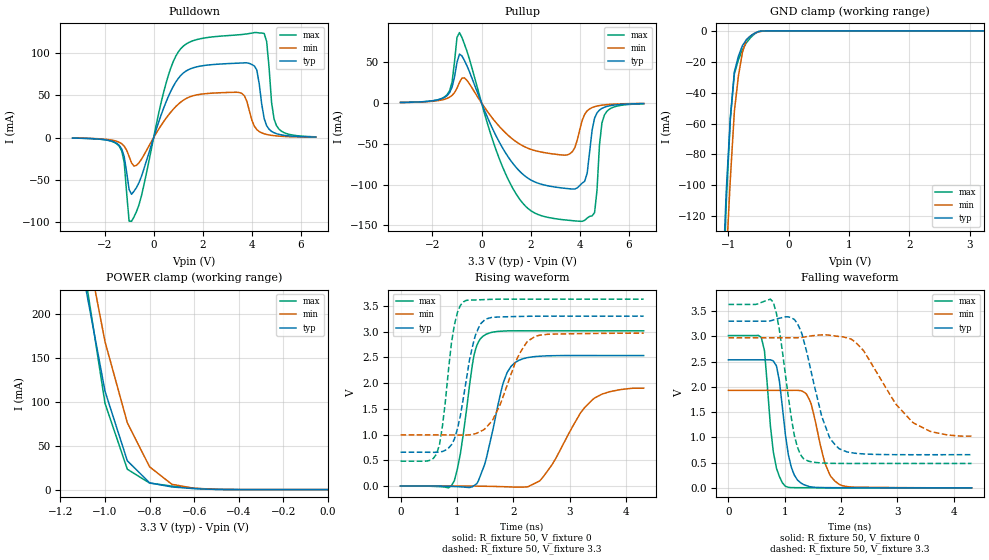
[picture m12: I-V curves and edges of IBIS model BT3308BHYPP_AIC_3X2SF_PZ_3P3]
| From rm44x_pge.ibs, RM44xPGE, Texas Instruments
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|   Model Cell BT3308BHYPP_AIC_3X2SF_PZ_3P3
|BT3308BHYPP_AIC_3X2SF_PZ_3P3
[Model]   BT3308BHYPP_AIC_3X2SF_PZ_3P3
Model_type   I/O
Polarity   Non-Inverting
Enable   Active-Low
Vinl =  1.15
Vinh =  1.55
Cref =  15.0001pF
Rref =  101.0000M
Vref =  0V
Vmeas =  1.65
C_comp   1.2p   1.2p   1.2p
[Model Spec]
Vinl   1.15   1.02   1.28
Vinh   1.55   1.45   1.65
[Temperature Range]   25   155   -40
[Voltage Range]   3.3   2.97   3.63
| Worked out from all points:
|   slope of the pulldown table from 0 to 0.495 V, typ, clamps not added: 11.9 ohm
|   slope of the pullup table from 0 to 0.495 V, typ, clamps not added: 14.3 ohm
|   GND clamp passes 1 mA (typ) near -0.53 V on its own axis
|   POWER clamp passes 1 mA (typ) near -0.59 V on its own axis
|   rising waveform, R_fixture 50, V_fixture 0: 20-80 % time 315ps typ, 599ps min, 226ps max; typ from 0 V to 2.53 V
|   rising waveform, R_fixture 50, V_fixture 3.3: 20-80 % time 265ps typ, 431ps min, 200ps max; typ from 0.657 V to 3.3 V
|   falling waveform, R_fixture 50, V_fixture 0: 20-80 % time 182ps typ, 257ps min, 153ps max; typ from 2.53 V to 0 V
|   falling waveform, R_fixture 50, V_fixture 3.3: 20-80 % time 362ps typ, 700ps min, 238ps max; typ from 3.3 V to 0.657 V
[POWER_clamp]
|   voltage   I(typ)   I(min)   I(max)
-3.3V     4.054A     4.63A      4.887A
-1.1V     248.3mA    301mA      262.7mA
-1.067V   202.9mA    256.9mA    207.9mA
-1.033V   157.5mA    212.7mA    153.1mA
-1V       112.1mA    168.6mA    98.29mA
-900mV    32.88mA    76.23mA    23.22mA
-800mV    7.705mA    25.95mA    7.475mA
-700mV    3.033mA    6.039mA    3.99mA
-600mV    1.087mA    1.528mA    1.425mA
-500mV    187uA      368.9uA    203.4uA
0V        443pA      6.158nA    417pA
[Pulldown]
|   voltage   I(typ)   I(min)   I(max)
-3.3V     -593uA     -522.6uA   -580.3uA
-1.4V     -9.188mA   -5.565mA   -10.35mA
-1.2V     -22.55mA   -10.08mA   -29.13mA
-1V       -61.66mA   -22.23mA   -99.07mA
-900mV    -67.21mA   -30.1mA    -99.29mA
1V        70.16mA    39.61mA    101.5mA
3.5V      88.44mA    53.41mA    122.1mA
4.2V      80.27mA    9.542mA    124.6mA
4.6V      14.18mA    3.749mA    114.2mA
4.8V      7.418mA    2.695mA    42.04mA
5V        4.687mA    2.03mA     14.29mA
6.6V      680.4uA    493.7uA    947.4uA
[Pullup]
|   voltage   I(typ)   I(min)   I(max)
-3.3V     671.9uA    618.2uA    613.1uA
-1.4V     9.171mA    5.687mA    10.35mA
-900mV    59.98mA    25.21mA    86.36mA
600mV     -40.93mA   -24.46mA   -58.45mA
1.4V      -78.76mA   -47.34mA   -111.2mA
3.5V      -105mA     -63.56mA   -143.7mA
4.1V      -98.16mA   -21.1mA    -145.1mA
4.3V      -85.91mA   -9.61mA    -141.1mA
4.6V      -18.69mA   -4.516mA   -134.6mA
4.8V      -8.691mA   -3.128mA   -51.49mA
5V        -5.242mA   -2.297mA   -14.81mA
6.6V      -711.8uA   -541.3uA   -921.2uA
[GND_clamp]
|   voltage   I(typ)   I(min)   I(max)
-3.3V     -3.25A     -2.875A    -4.945A
-1.1V     -166.9mA   -205mA     -187mA
-1.033V   -102.7mA   -146.7mA   -110.1mA
-966.7mV  -55.96mA   -95.69mA   -57.01mA
-900mV    -26.55mA   -52.03mA   -27.79mA
-833.3mV  -16.49mA   -29.28mA   -18.76mA
-766.7mV  -9.537mA   -13.91mA   -12.06mA
-700mV    -5.687mA   -5.923mA   -7.702mA
-566.7mV  -1.566mA   -1.63mA    -2.054mA
-500mV    -402.1uA   -594uA     -459.6uA
-366.7mV  -18.7uA    -59.22uA   -17.4uA
3.233V    423.5pA    4.09uA     323pA
[Ramp]
| variable   typ   min   max
dV/dt_f   1.638302/0.3729057n   1.223267/0.733161n   1.953849/0.2452135n
dV/dt_r   1.540285/0.3180453n   1.172218/0.6246788n   1.831658/0.2269715n
R_load = 50
[Rising Waveform]
R_fixture = 50
V_fixture = 0
V_fixture_min = 0
V_fixture_max = 0
|   time   V(typ)   V(min)   V(max)
0s        -4.976uV   -2.78uV    -6.755uV
956ps     -9.91mV    198.9uV    105mV
1.064ns   -15.38mV   128.6uV    636mV
1.304ns   7.149mV    -1.954mV   2.538V
1.492ns   414.2mV    -4.662mV   2.929V
1.82ns    1.995V     -12.79mV   3.009V
2.036ns   2.4V       -21.33mV   3.015V
2.472ns   2.521V     99.87mV    3.014V
3.444ns   2.534V     1.708V     3.014V
4.316ns   2.534V     1.9V       3.014V
[Rising Waveform]
R_fixture = 50
V_fixture = 3.3
V_fixture_min = 2.97
V_fixture_max = 3.63
|   time   V(typ)   V(min)   V(max)
0s        656.6mV    993.3mV    482.4mV
640ps     655.6mV    993.3mV    623.4mV
744ps     671mV      993.1mV    1.162V
956ps     911.4mV    990.3mV    3.129V
1.116ns   1.712V     987.9mV    3.576V
1.332ns   2.938V     1.017V     3.614V
1.52ns    3.244V     1.138V     3.622V
2.108ns   3.294V     2.562V     3.63V
2.4ns     3.298V     2.911V     3.63V
4.316ns   3.3V       2.969V     3.63V
[Falling Waveform]
R_fixture = 50
V_fixture = 0
V_fixture_min = 0
V_fixture_max = 0
|   time   V(typ)   V(min)   V(max)
0s        2.534V     1.93V      3.014V
584ps     2.533V     1.93V      2.975V
640ps     2.533V     1.93V      2.71V
852ps     2.415V     1.93V      389.6mV
1.012ns   1.045V     1.93V      30.07mV
1.224ns   156.7mV    1.93V      3.731mV
1.44ns    23.5mV     1.74V      1.968mV
1.712ns   5.245mV    492.9mV    537.2uV
1.964ns   2.809mV    70.58mV    297.7uV
4.316ns   94.61uV    817.4uV    5.461uV
[Falling Waveform]
R_fixture = 50
V_fixture = 3.3
V_fixture_min = 2.97
V_fixture_max = 3.63
|   time   V(typ)   V(min)   V(max)
0s        3.3V       2.97V      3.63V
796ps     3.322V     2.97V      3.674V
904ps     3.358V     2.97V      3.127V
1.168ns   3.334V     2.97V      1.044V
1.332ns   2.932V     2.983V     577.7mV
1.656ns   1.416V     3.027V     492.6mV
1.964ns   775.2mV    2.996V     483.1mV
2.4ns     671.5mV    2.713V     482.6mV
3.268ns   655.7mV    1.298V     482.5mV
4.316ns   656.5mV    1.023V     482.4mV
